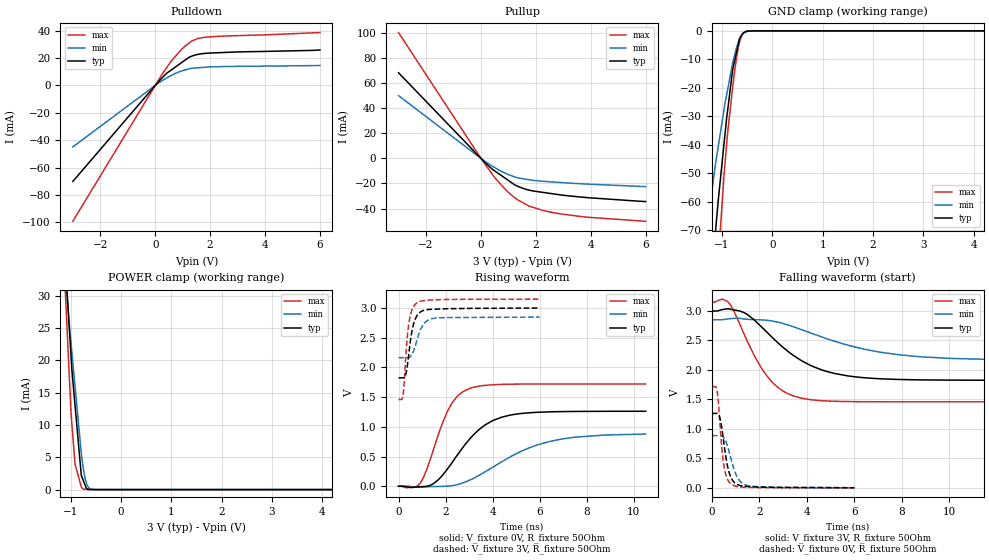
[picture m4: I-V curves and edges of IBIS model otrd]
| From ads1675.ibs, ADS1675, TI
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|   otrd Model
[Model]   otrd
Model_type   3-state
Polarity   Non-Inverting
Vmeas = 1.5
Vref = 0
Cref = 5pF
Rref = 500
|   typ   min   max
|   (nom PVT)   (Fast PVT)   (slow PVT)
|C_comp from frequency method(F=32MHz)
|Average
|C_comp   6.464e-12   5.452e-12   7.583e-12
|ON state : BUFFER OUTPUT TURNED HIGH
|C_comp   6.464e-12   5.452e-12   7.583e-12
|OFF state: BUFFER IN HIGH IMPEDANCE
C_comp   3.742e-12   2.938e-12   4.457e-12
|C_comp from L-C Tank method(L=1nH)
|ON state : BUFFER OUTPUT TURNED HIGH
|Resonant Frequency(Hz)   2.87e9   3.12e9   2.66e9
|C_comp   3.078e-12   2.605e-12   3.584e-12
|OFF state: BUFFER IN HIGH IMPEDANCE
|Resonant Frequency(Hz)   2.93e9   3.23e9   2.7e9
|C_comp   2.953e-12   2.43e-12   3.478e-12
| Where nom  PVT is Nominal Process,  3V,  51C
|   Fast PVT is Strong Process,   3.15V,  -40C
|   Slow PVT is Weak Process,   2.85V,  111C
[Voltage Range]   3   2.85   3.15
|Ambient Temperature   25   85   -40
|Junction Temperature
[Temperature Range]   51   111   -40
[Pullup Reference]   3   2.85   3.15
[Pulldown Reference]   0   0   0
[Power Clamp Reference]   3   2.85   3.15
[GND Clamp Reference]   0   0   0
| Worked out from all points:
|   slope of the pulldown table from 0 to 0.45 V, typ, clamps not added: 47.8 ohm
|   slope of the pullup table from 0 to 0.45 V, typ, clamps not added: 48.9 ohm
|   GND clamp passes 1 mA (typ) near -0.59 V on its own axis
|   POWER clamp passes 1 mA (typ) near -0.73 V on its own axis
|   falling waveform, V_fixture 3V, R_fixture 50Ohm: 20-80 % time 2.25ns typ, 3.49ns min, 1.39ns max; typ from 3 V to 1.82 V
|   rising waveform, V_fixture 0V, R_fixture 50Ohm: 20-80 % time 1.6ns typ, 2.57ns min, 986ps max; typ from 0 V to 1.26 V
|   rising waveform, V_fixture 3V, R_fixture 50Ohm: 20-80 % time 278ps typ, 376ps min, 218ps max; typ from 1.82 V to 3 V
|   falling waveform, V_fixture 0V, R_fixture 50Ohm: 20-80 % time 311ps typ, 418ps min, 232ps max; typ from 1.26 V to 0.001 V
[Pulldown]
|   Voltage   I(typ)   I(min)   I(max)
-3V       -70.2mA    -44.95mA   -99.32mA
242.5mV   5.395mA    3.388mA    8.009mA
420mV     8.976mA    5.561mA    13.13mA
614.2mV   11.76mA    7.657mA    18.56mA
1.093V    18.63mA    11.39mA    28.92mA
1.329V    21.43mA    12.55mA    32.51mA
1.553V    22.71mA    12.94mA    34.4mA
1.906V    23.64mA    13.46mA    35.44mA
6V        25.95mA    14.6mA     38.7mA
[GND Clamp]
|   Voltage   I(typ)   I(min)   I(max)
-3V       -479.3mA   -333.9mA   -693.5mA
-1.503V   -145.2mA   -96.89mA   -214.1mA
-1.206V   -86.11mA   -57.23mA   -120.9mA
-1.131V   -71.17mA   -47.23mA   -98.61mA
-1.062V   -57.54mA   -39.31mA   -77.99mA
-963.9mV  -40.62mA   -28.25mA   -51.96mA
-909mV    -31.11mA   -22.68mA   -40.34mA
-786mV    -13.55mA   -11.26mA   -19.61mA
-711.9mV  -7.665mA   -6.071mA   -9.727mA
-652.1mV  -2.913mA   -2.94mA    -4.097mA
-513.4mV  -197.2uA   -332.5uA   -139.7uA
6V        0A         0A         0A
[Pullup]
|   Voltage   I(typ)   I(min)   I(max)
-3V       68.19mA    49.98mA    100.2mA
0V        0A         0A         0A
420mV     -8.738mA   -6.297mA   -12.9mA
554.4mV   -10.79mA   -8.014mA   -16.64mA
957.6mV   -16.93mA   -12.54mA   -26.2mA
1.317V    -22mA      -15.4mA    -32.74mA
1.764V    -25.39mA   -17.07mA   -38.09mA
2.303V    -27.26mA   -18.33mA   -41.72mA
2.974V    -29.35mA   -19.36mA   -44.5mA
3.938V    -31.41mA   -20.58mA   -47mA
6V        -34.42mA   -22.53mA   -50.15mA
[POWER Clamp]
|   Voltage   I(typ)   I(min)   I(max)
-3V       208.2mA    183.4mA    247.3mA
-1.608V   97.95mA    84.02mA    114.7mA
-1.015V   23.79mA    24.76mA    15.92mA
-989.1mV  20.6mA     22.63mA    11.77mA
-972mV    18.47mA    21.2mA     10.08mA
-910.3mV  13.07mA    16.04mA    3.959mA
-786mV    2.198mA    5.624mA    416uA
-737.1mV  1.224mA    2.84mA     64.32uA
-701.1mV  506.5uA    1.454mA    38.88uA
-661.2mV  91.78uA    576.6uA    10.68uA
-561.5mV  7.578uA    35.55uA    1.333uA
6V        0A         0A         0A
[Ramp]
R_load = 50
|   typ   min   max
dV/dt_r   0.757701/1.60131e-09   0.531862/2.61163e-09   1.03249/9.82422e-10
dV/dt_f   0.705165/2.2501e-09   0.411202/3.51773e-09   1.0142/1.39323e-09
[Falling Waveform]
V_fixture = 3V
V_fixture_min = 2.85V
V_fixture_max = 3.15V
R_fixture = 50Ohm
|   Time   V(typ)   V(min)   V(max)
0s        3V         2.85V      3.15V
442ps     3.025V     2.852V     3.201V
709ps     3.037V     2.868V     3.141V
1.453ns   2.95V      2.861V     2.522V
2.294ns   2.65V      2.843V     1.912V
2.921ns   2.41V      2.796V     1.662V
3.704ns   2.175V     2.695V     1.528V
5.139ns   1.943V     2.49V      1.469V
7.826ns   1.839V     2.261V     1.46V
14.75ns   1.825V     2.167V     1.46V
[Rising Waveform]
V_fixture = 0V
V_fixture_min = 0V
V_fixture_max = 0V
R_fixture = 50Ohm
|   Time   V(typ)   V(min)   V(max)
0s        1.107nV    1.49nV     919.7pV
926ps     -7.196mV   -16.74mV   55.66mV
1.479ns   43.01mV    -4.073mV   610.7mV
2.171ns   339.8mV    5.268mV    1.33V
2.557ns   556.5mV    34.54mV    1.536V
3.051ns   807.3mV    108mV      1.65V
3.719ns   1.042V     252.1mV    1.699V
4.395ns   1.164V     414.9mV    1.715V
6.43ns    1.253V     754.9mV    1.721V
10.5ns    1.262V     879mV      1.721V
[Rising Waveform]
V_fixture = 3V
V_fixture_min = 2.85V
V_fixture_max = 3.15V
R_fixture = 50Ohm
|   Time   V(typ)   V(min)   V(max)
0s        1.825V     2.164V     1.46V
194ps     1.824V     2.165V     1.54V
240ps     1.831V     2.165V     1.734V
362ps     1.994V     2.163V     2.469V
477ps     2.362V     2.174V     2.829V
608ps     2.682V     2.249V     3.002V
787ps     2.874V     2.467V     3.089V
1.059ns   2.959V     2.726V     3.124V
1.401ns   2.979V     2.82V      3.137V
5.999ns   3V         2.848V     3.15V
[Falling Waveform]
V_fixture = 0V
V_fixture_min = 0V
V_fixture_max = 0V
R_fixture = 50Ohm
|   Time   V(typ)   V(min)   V(max)
0s        1.262V     886.5mV    1.72V
192ps     1.264V     886.2mV    1.697V
316ps     1.218V     887.5mV    1.23V
411ps     1.034V     883.3mV    704.5mV
509ps     751.1mV    849.4mV    370.4mV
650ps     384.5mV    715.3mV    154.2mV
822ps     162.2mV    469.6mV    61.06mV
1.105ns   49.94mV    157.2mV    19.43mV
1.462ns   24.79mV    42.17mV    9.203mV
5.999ns   994.2uV    3.137mV    63.34uV
